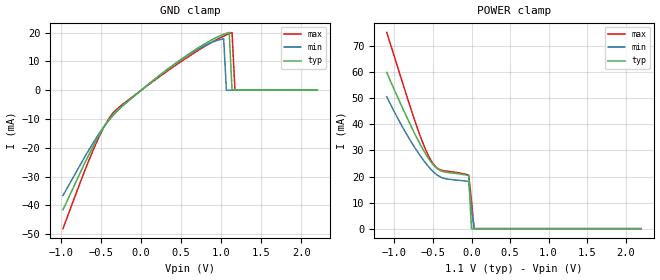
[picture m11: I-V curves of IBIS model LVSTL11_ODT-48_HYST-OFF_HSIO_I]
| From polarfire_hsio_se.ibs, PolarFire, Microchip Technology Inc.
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|   Model LVSTL11_ODT-48_HYST-OFF_HSIO_I
[Model]   LVSTL11_ODT-48_HYST-OFF_HSIO_I
Model_type   Input
Vinl =   0.083
Vinh =   0.283
|   typ   min   max
C_comp_pullup   1.335e-12   1.335e-12   1.380e-12
C_comp_pulldown  1.335e-12   1.335e-12   1.380e-12
[Temperature Range]  25C   100C   -40C
[Voltage Range]  1.1   1.045   1.155
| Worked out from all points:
|   GND clamp passes 1 mA (typ) near -0.04 V on its own axis
|   POWER clamp passes 1 mA (typ) near -0.00 V on its own axis
[GND Clamp]
| Voltage   I(typ)   I(min)   I(max)
-974.5mV  -41.51mA   -36.6mA    -48.12mA
-577.5mV  -18.37mA   -17.39mA   -19.5mA
-469.2mV  -13.11mA   -12.9mA    -13.1mA
-360.9mV  -8.942mA   -9.127mA   -8.294mA
378.1mV   8.229mA    8.214mA    7.621mA
928.1mV   18.13mA    17.09mA    17.32mA
1.031V    19.41mA    17.86mA    18.78mA
1.066V    19.76mA    0A         19.22mA
1.1V      20.08mA    0A         19.63mA
1.136V    0A         0A         20.03mA
1.172V    0A         0A         0A
2.2V      0A         0A         0A
[POWER Clamp]
| Voltage   I(typ)   I(min)   I(max)
-1.1V     59.95mA    50.61mA    75.31mA
-902.3mV  46.77mA    39.36mA    56.69mA
-721.9mV  35.56mA    30.46mA    40.24mA
-613.6mV  29.59mA    25.87mA    31.59mA
-541.4mV  26.22mA    23.24mA    26.98mA
-469.2mV  23.65mA    21.13mA    23.88mA
-397mV    22.17mA    19.73mA    22.48mA
-288.8mV  21.48mA    18.92mA    21.94mA
-36.09mV  20.36mA    18.11mA    20.55mA
0V        0A         7.218mA    10.68mA
34.38mV   0A         0A         0A
2.2V      0A         0A         0A
